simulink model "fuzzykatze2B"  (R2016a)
settings: Solver=ode45  StartTime=0.0  StopTime=100  RelTol=1e-5
undefined symbols (not defined in the file or in its folder): p
libraries: libregler2 x4

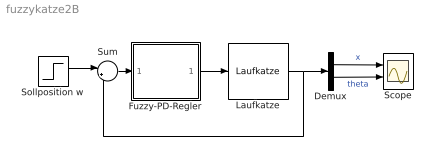
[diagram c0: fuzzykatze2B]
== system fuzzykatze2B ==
  Demux : Demux  Outputs=2
  Fuzzy-PD-Regler : Subsystem
  Laufkatze : libregler2/Laufkatze  mk=100  ml=500  l=3  g=9.81
  Scope : Scope  NumInputPorts=2
  Sollposition w : Step  Time=5  Before=[0,0]  After=[10,0]  SampleTime=0
  Sum : Sum  Inputs=|+-
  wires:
  Fuzzy-PD-Regler/1(u) -> Laufkatze/1
  Demux/1 -> Scope/1  "x"
  Demux/2 -> Scope/2  "theta"
  Laufkatze/1 -> Demux/1, Sum/2
  Sollposition w/1 -> Sum/1
  Sum/1 -> Fuzzy-PD-Regler/1(e)

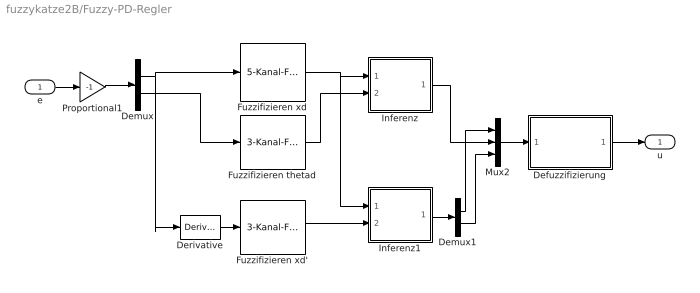
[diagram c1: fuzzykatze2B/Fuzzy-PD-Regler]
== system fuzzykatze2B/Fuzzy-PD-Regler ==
  e : Inport
  Defuzzifizierung : Subsystem
  Demux : Demux  Outputs=2
  Demux1 : Demux  Outputs=2
  Derivative : Derivative
  Fuzzifizieren thetad : libregler2/3-Kanal-Fuzzifizierer  SystemSampleTime=-1  w=bth  offset=0
  Fuzzifizieren xd : libregler2/5-Kanal-Fuzzifizierer  SystemSampleTime=-1  w=bx  offset=0
  Fuzzifizieren xd' : libregler2/3-Kanal-Fuzzifizierer  SystemSampleTime=-1  w=bv  offset=0
  Inferenz : Subsystem
  Inferenz1 : Subsystem
  Mux2 : Mux  Inputs=3
  Proportional1 : Gain  Gain=-1
  u : Outport
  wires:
  Fuzzifizieren xd/1 -> Inferenz/1(E1), Inferenz1/1(E1)
  Demux/1 -> Derivative/1, Fuzzifizieren xd/1
  Demux/2 -> Fuzzifizieren thetad/1
  e/1 -> Proportional1/1
  Derivative/1 -> Fuzzifizieren xd'/1
  Inferenz/1(u) -> Mux2/2
  Defuzzifizierung/1(sharp) -> u/1
  Mux2/1 -> Defuzzifizierung/1(fuzzy)
  Proportional1/1 -> Demux/1
  Inferenz1/1(u) -> Demux1/1
  Demux1/1 -> Mux2/1
  Demux1/2 -> Mux2/3
  Fuzzifizieren thetad/1 -> Inferenz/2(E2)
  Fuzzifizieren xd'/1 -> Inferenz1/2(E2)

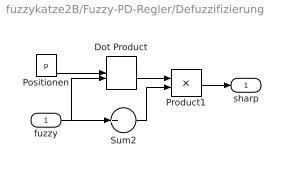
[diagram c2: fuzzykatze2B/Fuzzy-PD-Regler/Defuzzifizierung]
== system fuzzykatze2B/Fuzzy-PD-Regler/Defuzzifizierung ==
  fuzzy : Inport
  Dot Product : DotProduct
  Positionen : Constant  Value=p
  Product1 : Product  Inputs=*/
  Sum2 : Sum  Inputs=+
  sharp : Outport
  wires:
  Product1/1 -> sharp/1
  Sum2/1 -> Product1/2
  Positionen/1 -> Dot Product/1
  fuzzy/1 -> Dot Product/2, Sum2/1
  Dot Product/1 -> Product1/1

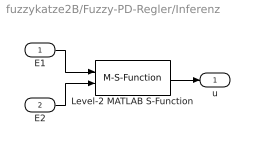
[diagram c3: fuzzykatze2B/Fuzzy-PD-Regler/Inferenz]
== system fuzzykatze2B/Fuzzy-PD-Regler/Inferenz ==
  E1 : Inport
  E2 : Inport  Port=2
  Level-2 MATLAB S-Function : M-S-Function  FunctionName=sfun_inferenz  Parameters=M
  u : Outport
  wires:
  Level-2 MATLAB S-Function/1 -> u/1
  E2/1 -> Level-2 MATLAB S-Function/2
  E1/1 -> Level-2 MATLAB S-Function/1

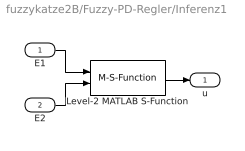
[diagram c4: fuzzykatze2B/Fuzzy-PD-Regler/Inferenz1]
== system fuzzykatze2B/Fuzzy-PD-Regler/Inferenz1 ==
  E1 : Inport
  E2 : Inport  Port=2
  Level-2 MATLAB S-Function : M-S-Function  FunctionName=sfun_inferenz  Parameters=M
  u : Outport
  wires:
  Level-2 MATLAB S-Function/1 -> u/1
  E2/1 -> Level-2 MATLAB S-Function/2
  E1/1 -> Level-2 MATLAB S-Function/1
